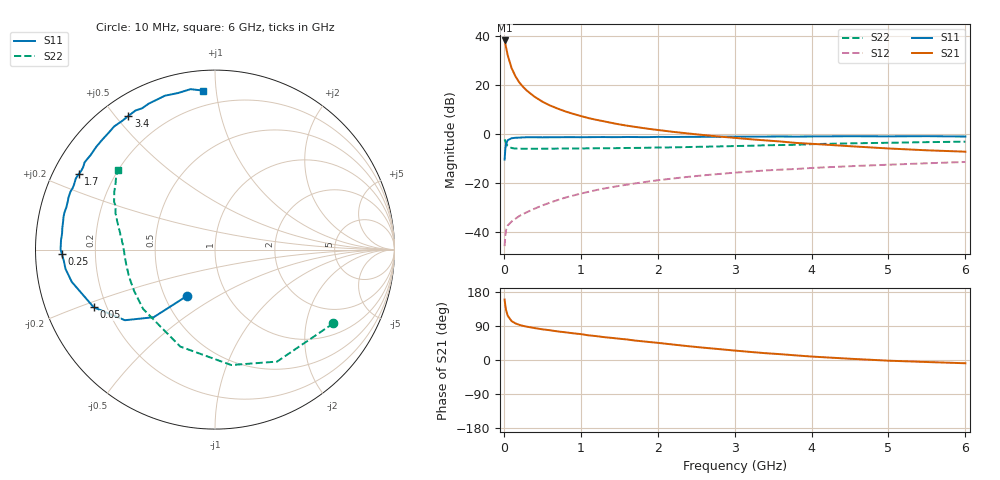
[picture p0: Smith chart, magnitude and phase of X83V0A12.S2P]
! SIEMENS Small Signal Semiconductors
! BFP136W
! Si NPN RF Bipolar Junction Transistor in SOT343
! VCE = 3 V  IC = 120 mA
! Common Emitter S-Parameters:  September  1994
# GHz  S  MA  R  50
!  f  S11  S21  S12  S22
! GHz  MAG  ANG  MAG  ANG  MAG  ANG  MAG  ANG
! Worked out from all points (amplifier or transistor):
!   40 points, 10 MHz to 6 GHz, reference 50 ohm
!   highest |S21| = 38.1 dB at 10 MHz (marker M1)
!   |S21| within 3 dB of that: start of sweep to 30.13 MHz
!   unconditionally stable (mu >= 1): 482.2 MHz to 2.899 GHz
!   at 200 MHz: K = 0.72, MSG = 27.2 dB, |S12| = -33.4 dB
!   at 1.5 GHz: K = 1.11, MAG = 10.6 dB, |S12| = -21.1 dB
!   at 6 GHz: K = 0.97, MSG = 2.1 dB, |S12| = -11.4 dB
!   S11 on the Smith chart (normalised r, x): 10 MHz: 0.65, -0.37; 50 MHz: 0.15, -0.22; 250 MHz: 0.08, -0.01; 1.7 GHz: 0.08, +0.26; 3.4 GHz: 0.08, +0.54; 6 GHz: 0.11, +0.92
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0.01  0.3011 -121.1  80.5 159.5  0.0052 67.5  0.7772 -31.9
0.02  0.5085 -132.2  68.37 142.6  0.0089 55.4  0.7134 -61.0
0.03  0.6377 -141.9  57.12 130.9  0.0113 49.1  0.6495 -82.0
0.05  0.7485 -154.6  40.35 116.9  0.0137 39.3  0.5739 -109.7
0.1  0.8181 -167.3  22.16 102.8  0.0165 38.0  0.5194 -140.5
0.15  0.84 -172.7  15.05 96.7  0.0188 41.2  0.506 -153.0
0.2  0.8444 -175.7  11.3 92.9  0.0213 43.7  0.5021 -159.7
0.25  0.8539 -178.4  9.116 90.0  0.0235 46.7  0.5016 -164.0
0.3  0.8603 179.9  7.629 87.9  0.0256 49.4  0.5005 -166.9
0.4  0.8596 176.5  5.743 84.2  0.0302 53.3  0.5016 -170.8
0.5  0.8567 174.0  4.577 81.0  0.0351 56.2  0.5027 -173.6
0.6  0.8591 172.0  3.818 78.5  0.0401 58.5  0.5038 -175.3
0.7  0.8605 169.6  3.295 75.4  0.0452 60.3  0.5048 -176.6
0.9  0.8639 166.1  2.579 70.5  0.0557 61.0  0.5068 -179.2
1.1  0.8632 161.8  2.111 65.1  0.0664 61.7  0.5106 179.2
1.7  0.8684 151.1  1.404 51.4  0.0983 59.3  0.5212 174.2
2.2  0.8705 142.8  1.108 40.8  0.1243 55.5  0.535 170.5
3.2  0.8841 126.0  0.784 21.4  0.1719 45.8  0.5773 161.7
3.4  0.8873 122.9  0.742 18.0  0.1812 43.7  0.5902 160.0
4.5  0.9017 108.0  0.565 3.3  0.2211 33.4  0.6462 150.3
5.5  0.9042 98.7  0.466 -5.3  0.2537 25.5  0.6838 143.7
6  0.8889 94.4  0.437 -8.6  0.2699 21.1  0.6985 140.8
